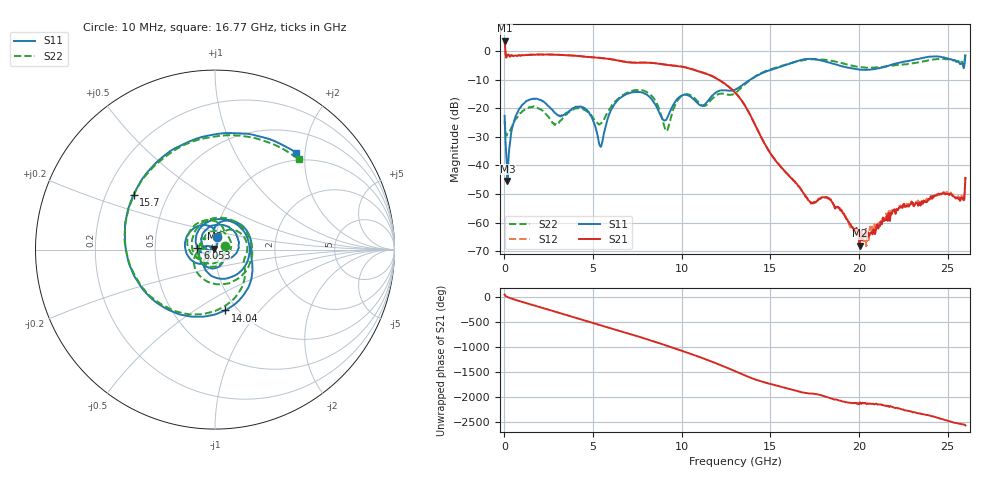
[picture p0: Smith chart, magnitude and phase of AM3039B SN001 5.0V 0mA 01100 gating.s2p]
!Agilent Technologies,E8364B,MY43040894,A.07.50.67
!Agilent E8364B: A.07.50.67
!Date: Tuesday, June 28, 2016 08:06:16
!Correction: S11(Full 2 Port(1,2))
!S21(Full 2 Port(1,2))
!S12(Full 2 Port(1,2))
!S22(Full 2 Port(1,2))
!S2P File: Measurements: S11, S21, S12, S22:
# Hz S  dB  R 50
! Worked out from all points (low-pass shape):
!   1601 points, 10 MHz to 26 GHz, reference 50 ohm
!   highest |S21| = 3.65 dB at 10 MHz (marker M1); lowest = -68.0 dB at 20.04 GHz (marker M2)
!   |S21| within 3 dB of the highest: start of sweep to 44.31 MHz
!   lowest |S11| = -45.4 dB at 172.4 MHz (marker M3), VSWR 1.01, Z = 49.7 + j0.447 ohm
!   |S11| at or under -10 dB: start of sweep to 13.85 GHz
!   |S22| runs from -29.6 to -1.0 dB; largest |S21 - S12| = 0.026
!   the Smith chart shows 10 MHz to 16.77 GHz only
!   S11 on the Smith chart (normalised r, x): 10 MHz: 1.02, +0.15; 6.053 GHz: 0.82, +0.02; 14.04 GHz: 0.88, -0.67; 15.7 GHz: 0.32, +0.28; 16.77 GHz: 0.85, +1.82
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1e7  -22.63 79.6  3.65 40.7  3.72 41.6  -24.55 17.5
1.724375e8  -45.38 123.3  -1.26 -8.4  -1.20 -8.2  -28.61 -59.5
1.650619e9  -16.61 57.3  -1.26 -173.1  -1.21 -173.0  -19.33 61.2
2.673975e9  -20.35 -31.0  -1.25 81.0  -1.18 81.2  -24.70 -29.9
3.486162e9  -21.65 -57.5  -1.45 -3.4  -1.40 -3.2  -22.24 -57.3
4.347081e9  -19.56 -130.5  -1.84 -93.8  -1.80 -93.6  -20.14 -156.0
5.175512e9  -27.47 152.0  -2.29 179.1  -2.24 179.3  -24.75 54.9
6.052675e9  -20.10 174.5  -2.89 84.2  -2.84 84.5  -18.98 -157.2
7.628319e9  -14.33 -18.8  -4.04 -80.9  -3.98 -80.7  -13.55 -33.1
8.684162e9  -20.81 -133.8  -4.40 159.9  -4.34 160.1  -19.51 -169.0
9.951175e9  -15.70 -179.3  -5.40 11.7  -5.32 11.8  -15.92 165.0
1.3005e10  -13.52 -14.4  -14.47 -39.6  -14.43 -40.0  -14.74 -27.4
1.40446e10  -9.28 -80.5  -24.59 167.0  -24.54 166.3  -9.27 -91.1
1.570146e10  -5.23 146.0  -41.23 -0.1  -41.13 0.6  -5.02 136.7
1.677355e10  -3.05 50.2  -48.78 -99.6  -48.70 -98.1  -3.27 47.2
1.734208e10  -2.74 -6.6  -53.10 -126.0  -52.96 -126.5  -2.88 -3.0
1.838168e10  -4.15 -104.3  -51.79 141.8  -52.02 141.5  -3.32 -94.2
2.003854e10  -6.52 127.3  -68.04 50.2  -63.09 40.7  -5.58 137.0
2.167916e10  -5.04 16.5  -56.65 -21.1  -55.97 -18.1  -5.25 22.2
2.31411e10  -2.97 -93.1  -53.69 -137.9  -52.73 -144.2  -4.15 -83.7
2.422943e10  -1.87 178.4  -50.83 133.3  -50.27 135.6  -2.92 -166.6
2.6e10  -1.64 -21.1  -44.38 -39.3  -44.10 -39.8  -0.97 8.4
